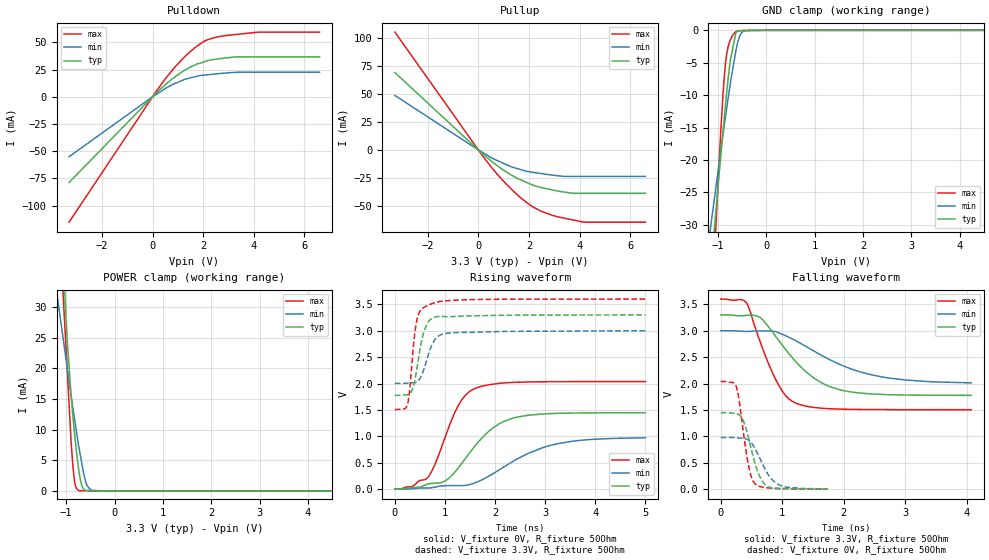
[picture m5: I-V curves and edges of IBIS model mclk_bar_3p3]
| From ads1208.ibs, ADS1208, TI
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|   mclk_bar_3p3 Model
[Model]   mclk_bar_3p3
Model_type   I/O
Polarity   Non-Inverting
Enable   Active-Low
Vinl = 0.99
Vinh = 2.31
Vmeas = 1.65
Vref = 1.65
Cref = 30pF
Rref = 50
|   typ   min   max
|   (nom PVT)   (fast PVT)   (slow PVT)
|C_comp from frequency sweep method (F=10MHz)
|Average
|C_comp   1.932e-12   1.849e-12   1.992e-12
|ON state : BUFFER OUTPUT TURNED HIGH
C_comp   2.228e-12   2.216e-12   2.229e-12
|OFF state: BUFFER IN HIGH IMPEDANCE
|C_comp   1.635e-12   1.482e-12   1.754e-12
|C_comp from LC tank measurement(L=1nH)
|Average
|Resonant Frequency(Hz)   5.515e+09   5.640e+09   4.685e+09
|C_comp   8.356e-13   7.979e-13   1.157e-12
|ON state : BUFFER OUTPUT TURNED HIGH
|Resonant Frequency(Hz)   5.670e+09   5.740e+09   4.780e+09
|C_comp   7.887e-13   7.696e-13   1.110e-12
|OFF state: BUFFER IN HIGH IMPEDANCE
|Resonant Frequency(Hz)   5.360e+09   5.540e+09   4.590e+09
|C_comp   8.826e-13   8.261e-13   1.204e-12
| Where nom  PVT is Nominal Process, 3.3V, 35C
|   Fast PVT is Strong Process,  3.6V, -40C
|   Slow PVT is Weak Process,   3V, 95C
[Model Spec]
|Subparameter   typ   min   max
Vinh   2.31   2.1   2.52
Vinl   0.99   0.9   1.08
[Voltage Range]   3.3   3   3.6
|Ambient Temperature   25   85   -40
|Junction Temperature
[Temperature Range]   35   95   -40
[Pullup Reference]   3.3   3   3.6
[Pulldown Reference]   0   0   0
[Power Clamp Reference]   3.3   3   3.6
[GND Clamp Reference]   0   0   0
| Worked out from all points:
|   slope of the pulldown table from 0 to 0.495 V, typ, clamps not added: 45.6 ohm
|   slope of the pullup table from 0 to 0.495 V, typ, clamps not added: 51.4 ohm
|   GND clamp passes 1 mA (typ) near -0.64 V on its own axis
|   POWER clamp passes 1 mA (typ) near -0.68 V on its own axis
|   falling waveform, V_fixture 3.3V, R_fixture 50Ohm: 20-80 % time 718ps typ, 1.07ns min, 439ps max; typ from 3.3 V to 1.78 V
|   rising waveform, V_fixture 0V, R_fixture 50Ohm: 20-80 % time 793ps typ, 1.16ns min, 526ps max; typ from 0 V to 1.45 V
|   rising waveform, V_fixture 3.3V, R_fixture 50Ohm: 20-80 % time 181ps typ, 224ps min, 135ps max; typ from 1.78 V to 3.3 V
|   falling waveform, V_fixture 0V, R_fixture 50Ohm: 20-80 % time 206ps typ, 269ps min, 153ps max; typ from 1.45 V to 0.005 V
[Pulldown]
|   Voltage   I(typ)   I(min)   I(max)
-3.3V     -78.72mA   -55.04mA   -115.2mA
172.8mV   4.011mA    2.634mA    5.902mA
633.6mV   13.71mA    9.355mA    20.31mA
939.6mV   19.26mA    12.76mA    28.74mA
1.399V    26.15mA    16.85mA    39.61mA
1.706V    29.38mA    18.61mA    45.77mA
2.167V    33.27mA    20.21mA    52.41mA
2.934V    35.75mA    21.95mA    56.39mA
3.28V     36.64mA    22.47mA    57.23mA
4.162V    36.64mA    22.6mA     59.37mA
6.6V      36.64mA    22.6mA     59.45mA
[GND Clamp]
|   Voltage   I(typ)   I(min)   I(max)
-3.3V     -235.4mA   -157.4mA   -409mA
-1.175V   -39.61mA   -31.77mA   -51.02mA
-1.105V   -33.49mA   -27.86mA   -40.02mA
-1.02V    -26.07mA   -23.06mA   -27.12mA
-896.4mV  -15.76mA   -16.2mA    -10.22mA
-817.2mV  -9.617mA   -12.02mA   -3.648mA
-745.8mV  -4.749mA   -8.387mA   -1.548mA
-627mV    -394uA     -3.141mA   -216.8uA
-583.2mV  -105.4uA   -1.716mA   -71.23uA
-510mV    -85.17uA   -360.4uA   -35.45uA
-285mV    -47.35uA   -475.6nA   -422.2nA
6.6V      0A         0A         0A
[Pullup]
|   Voltage   I(typ)   I(min)   I(max)
-3.3V     69.39mA    48.86mA    105.7mA
18mV      -367.3uA   -262.1uA   -572.9uA
478.8mV   -9.331mA   -6.5mA     -14.46mA
939.6mV   -17.23mA   -11.47mA   -26.71mA
1.246V    -21.7mA    -14.53mA   -33.9mA
1.706V    -27.17mA   -17.83mA   -43.57mA
2.012V    -30.17mA   -19.5mA    -48.9mA
2.473V    -33.62mA   -21.14mA   -54.88mA
2.927V    -35.88mA   -22.58mA   -58.65mA
3.703V    -38.72mA   -23.74mA   -62.6mA
4.162V    -38.9mA    -23.74mA   -64.76mA
6.6V      -38.9mA    -23.74mA   -64.76mA
[POWER Clamp]
|   Voltage   I(typ)   I(min)   I(max)
-3.3V     1.095A     159.9mA    409.3mA
-1.224V   84.63mA    34.18mA    57.65mA
-1.158V   62.94mA    30.29mA    46.91mA
-1.094V   45.66mA    26.65mA    36.5mA
-1.036V   33.48mA    23.35mA    28.05mA
-896.4mV  15.35mA    15.4mA     7.754mA
-856.8mV  11.78mA    13.25mA    3.618mA
-820.8mV  8.85mA     11.39mA    1.239mA
-734.4mV  3.123mA    7.034mA    31uA
-646.8mV  341.7uA    3.16mA     20.07uA
-486mV    61.03uA    96.96uA    0A
6.6V      0A         0A         0A
[Ramp]
R_load = 50
|   typ   min   max
dV/dt_r   0.868534/7.89549e-10   0.58355/1.15033e-09   1.22229/5.21242e-10
dV/dt_f   0.914217/7.1624e-10   0.596741/1.08251e-09   1.25642/4.37283e-10
[Falling Waveform]
V_fixture = 3.3V
V_fixture_min = 3V
V_fixture_max = 3.6V
R_fixture = 50Ohm
|   Time   V(typ)   V(min)   V(max)
0s        3.3V       3V         3.6V
422ps     3.29V      2.987V     3.523V
643ps     3.25V      2.996V     2.784V
897ps     2.888V     2.983V     2.067V
1.068ns   2.626V     2.899V     1.756V
1.238ns   2.392V     2.8V       1.621V
1.627ns   2.023V     2.542V     1.535V
2.07ns    1.85V      2.298V     1.513V
2.713ns   1.791V     2.108V     1.507V
4.07ns    1.777V     2.014V     1.506V
[Rising Waveform]
V_fixture = 0V
V_fixture_min = 0V
V_fixture_max = 0V
R_fixture = 50Ohm
|   Time   V(typ)   V(min)   V(max)
0s        687.8pV    1.217nV    632.9pV
349ps     31.06mV    8.08mV     52.35mV
667ps     99.34mV    22.4mV     233.6mV
1.006ns   157.6mV    65.58mV    993.6mV
1.255ns   389.1mV    66mV       1.566V
1.599ns   819.2mV    119.3mV    1.908V
2.06ns    1.225V     351.9mV    2.001V
2.457ns   1.368V     579.7mV    2.025V
3.266ns   1.436V     864.3mV    2.036V
4.999ns   1.448V     972.6mV    2.037V
[Rising Waveform]
V_fixture = 3.3V
V_fixture_min = 3V
V_fixture_max = 3.6V
R_fixture = 50Ohm
|   Time   V(typ)   V(min)   V(max)
0s        1.776V     2.003V     1.506V
251ps     1.791V     2.008V     1.597V
298ps     1.808V     2.012V     1.907V
368ps     1.939V     2.014V     2.689V
442ps     2.295V     2.034V     3.215V
555ps     2.896V     2.208V     3.426V
700ps     3.204V     2.643V     3.498V
858ps     3.269V     2.892V     3.547V
1.091ns   3.267V     2.958V     3.572V
4.999ns   3.3V       3V         3.6V
[Falling Waveform]
V_fixture = 0V
V_fixture_min = 0V
V_fixture_max = 0V
R_fixture = 50Ohm
|   Time   V(typ)   V(min)   V(max)
0s        1.448V     978.5mV    2.037V
254ps     1.429V     974.1mV    1.939V
299ps     1.409V     968.9mV    1.687V
362ps     1.311V     965.8mV    1.139V
447ps     994.9mV    933.4mV    476.5mV
503ps     724.8mV    870.4mV    217.2mV
558ps     479.7mV    769.8mV    103.4mV
707ps     104.7mV    410.7mV    34.11mV
921ps     15.38mV    100.9mV    14.77mV
1.741ns   4.617mV    6.367mV    1.436mV
